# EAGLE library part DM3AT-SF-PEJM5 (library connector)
CONN MICRO SD R/A PUSH-PUSH SMD
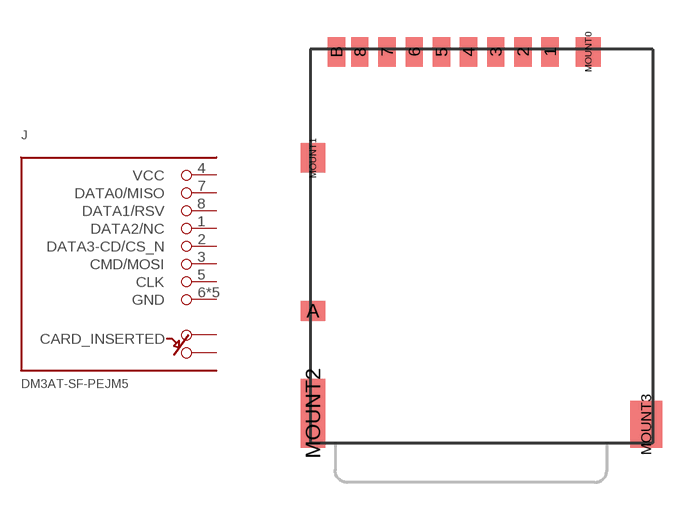
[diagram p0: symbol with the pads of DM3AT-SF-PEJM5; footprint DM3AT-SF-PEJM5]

Designator prefix J

## DM3AT-SF-PEJM5 (DESCRIPTION: CONN MICRO SD CARD PUSH-PUSH R/A; DIGIKEY: HR1964CT-ND; MANUFACTURER: Hirose Electric Co Ltd; MPN: DM3AT-SF-PEJM5)  [DM3AT-SF-PEJM5]
1  DATA2/NC
2  DATA3-CD/CS_N
3  CMD/MOSI
4  VCC
5  CLK
6  GND
7  DATA0/MISO
8  DATA1/RSV
A  A
B  B
MOUNT0  GND
MOUNT1  GND
MOUNT2  GND
MOUNT3  GND

## Footprint DM3AT-SF-PEJM5 (pad centres in mm)
Micro SD card holder with push-to-eject feature.
smd 0.7 x 1.2: 1 3.2,-0.1; 2 2.1,-0.1; 3 1,-0.1; 4 -0.1,-0.1; 5 -1.2,-0.1; 6 -2.3,-0.1; 7 -3.4,-0.1; 8 -4.5,-0.1; B -5.45,-0.1
smd 1 x 0.8: A -6.4,-10.6
smd 1 x 1.2: MOUNT0 4.75,-0.1; MOUNT1 -6.4,-4.4
smd 1 x 2.8: MOUNT2 -6.4,-14.75
smd 1.3 x 1.9: MOUNT3 7.1,-15.2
